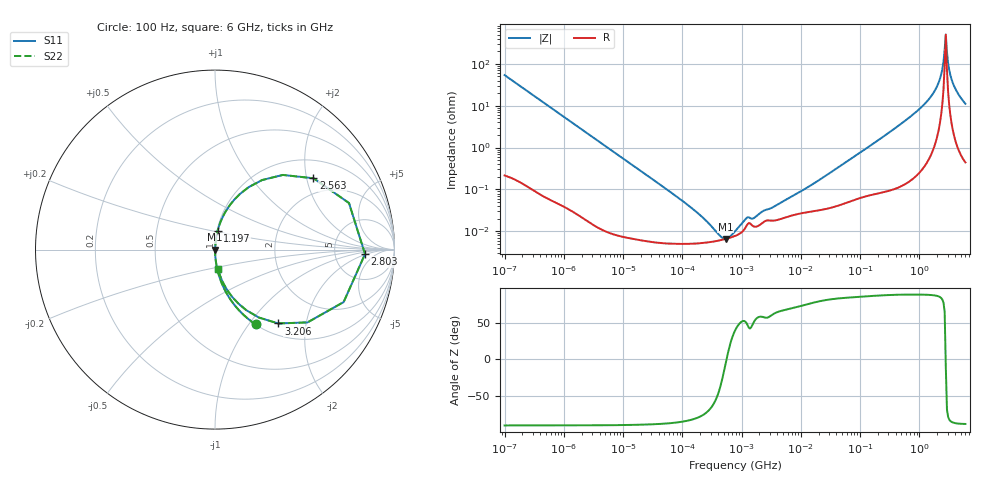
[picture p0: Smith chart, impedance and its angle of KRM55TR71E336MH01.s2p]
!Murata Part Number: KRM55TR71E336MH01
!These Parameters are Measured in Series Mode Connection
!Data Generated on Jan 08, 2026
!  o--ll--o
!Port1  Port2
!  o------o
!Operation Temp=25[degC], DC Bias Voltage=0[V]
!Freq. Start=100[Hz] Stop=6[GHz] 401[Steps]
# Hz S RI R 50
!Freq.(Hz) S11(Real) S11(Imag) S21(Real) S21(Imag) S12(Real) S12(Imag) S22(Real) S22(Imag)
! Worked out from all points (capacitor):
!   401 points, 100 Hz to 6 GHz, reference 50 ohm
!   read as one part in series: C = 29.4 uF near 109 Hz
!   lowest |Z| = 6.61 mohm at 541.4 kHz (marker M1)
!   series resonance near 556.9 kHz, so ESL is about 2.8 nH
!   S11 on the Smith chart (normalised r, x): 100 Hz: 1.00, -1.08; 1.197 GHz: 1.01, +0.21; 2.563 GHz: 1.50, +2.20; 2.803 GHz: 11, -2; 3.206 GHz: 1.20, -1.40; 6 GHz: 1.01, -0.22
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100  0.2269 -0.4168  0.7731 0.4168  0.7731 0.4168  0.2269 -0.4168
280  0.0371 -0.1863  0.9629 0.1863  0.9629 0.1863  0.0371 -0.1863
2008  0.000954 -0.0272  0.999 0.0272  0.999 0.0272  0.000954 -0.0272
40335  5.48e-05 -0.00136  0.9999 0.00136  0.9999 0.00136  5.48e-05 -0.00136
161617  5.1e-05 -0.00031  0.9999 0.00031  0.9999 0.00031  5.1e-05 -0.00031
361830  5.8e-05 -8.53e-05  0.9999 8.53e-05  0.9999 8.53e-05  5.8e-05 -8.53e-05
541393  6.59e-05 -5.3e-06  0.9999 5.3e-06  0.9999 5.3e-06  6.59e-05 -5.3e-06
774597  7.74e-05 6.31e-05  0.9999 -6.31e-05  0.9999 -6.31e-05  7.74e-05 6.31e-05
1212075  0.000135 0.000158  0.9999 -0.000158  0.9999 -0.000158  0.000135 0.000158
1658239  0.000129 0.000169  0.9999 -0.000169  0.9999 -0.000169  0.000129 0.000169
1.555665e7  0.0003 0.00128  0.9997 -0.00128  0.9997 -0.00128  0.0003 0.00128
3.124326e8  0.00147 0.0231  0.9985 -0.0231  0.9985 -0.0231  0.00147 0.0231
1.197065e9  0.0144 0.104  0.9856 -0.104  0.9856 -0.104  0.0144 0.104
2.048624e9  0.1062 0.2769  0.8938 -0.2769  0.8938 -0.2769  0.1062 0.2769
2.34314e9  0.2623 0.3874  0.7377 -0.3874  0.7377 -0.3874  0.2623 0.3874
2.562649e9  0.5486 0.3974  0.4514 -0.3974  0.4514 -0.3974  0.5486 0.3974
2.802721e9  0.8358 -0.0249  0.1642 0.0249  0.1642 0.0249  0.8358 -0.0249
3.065283e9  0.5155 -0.4056  0.4845 0.4056  0.4845 0.4056  0.5155 -0.4056
3.205649e9  0.3526 -0.4115  0.6474 0.4115  0.6474 0.4115  0.3526 -0.4115
3.505958e9  0.1749 -0.338  0.8251 0.338  0.8251 0.338  0.1749 -0.338
3.8344e9  0.0988 -0.267  0.9012 0.267  0.9012 0.267  0.0988 -0.267
6e9  0.0165 -0.109  0.9835 0.109  0.9835 0.109  0.0165 -0.109
